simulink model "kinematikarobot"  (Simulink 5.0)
settings: Solver=ode45  StartTime=0.0  StopTime=10.0  RelTol=1e-3

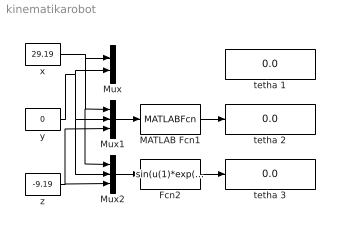
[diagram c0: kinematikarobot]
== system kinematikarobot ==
  Fcn2 : Fcn  Expr=sin(u(1)*exp(2.3*(-u(2))))
  MATLAB Fcn1 : MATLABFcn  MATLABFcn=fungsi1
  Mux : Mux  Inputs=2
  Mux1 : Mux  Inputs=3
  Mux2 : Mux  Inputs=3
  tetha 1 : Display
  tetha 2 : Display
  tetha 3 : Display
  x : Constant  Value=29.19
  y : Constant  Value=0
  z : Constant  Value=-9.19
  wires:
  x/1 -> Mux/1, Mux2/1, Mux1/1
  Mux/1 -> ?
  ? -> tetha 1/1
  y/1 -> Mux/2, Mux1/2, Mux2/2
  Mux1/1 -> MATLAB Fcn1/1
  MATLAB Fcn1/1 -> tetha 2/1
  Fcn2/1 -> tetha 3/1
  Mux2/1 -> Fcn2/1
  z/1 -> Mux2/3, Mux1/3
